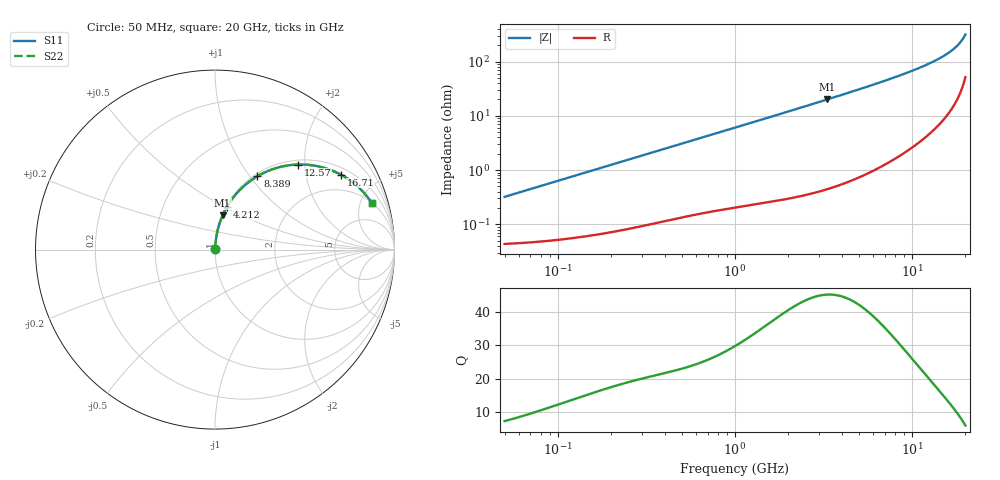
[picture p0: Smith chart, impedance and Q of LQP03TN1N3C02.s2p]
!Murata Part Number: LQP03TN1N3C02
!These Parameters are Measured in Series Mode Connection
!  o--[Z]--o
!Port1  Port2
!  o-------o
!Freq. Start=50[MHz] Stop=20[GHz], 401[Steps]
# Hz S RI R 50
!Freq.(Hz) S11(Real) S11(Imag) S21(Real) S21(Imag) S12(Real) S12(Imag) S22(Real) S22(Imag)
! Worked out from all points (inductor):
!   401 points, 50 MHz to 20 GHz, reference 50 ohm
!   read as one part in series: L = 1.01 nH near 51.52 MHz
!   highest Q = 45.1 at 3.314 GHz (marker M1), where L = 961 pH
!   S11 on the Smith chart (normalised r, x): 50 MHz: 1.00, +0.01; 4.212 GHz: 1.01, +0.51; 8.389 GHz: 1.04, +1.09; 12.57 GHz: 1.09, +1.85; 16.71 GHz: 1.27, +3.17; 20 GHz: 2.03, +6.23
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5e7  0.000445 0.00318  0.9996 -0.00318  0.9996 -0.00318  0.000445 0.00318
1.364002e8  0.00066 0.00858  0.9993 -0.00858  0.9993 -0.00858  0.00066 0.00858
3.721004e8  0.00161 0.0229  0.9984 -0.0229  0.9984 -0.0229  0.00161 0.0229
6.380365e8  0.00307 0.0387  0.9969 -0.0387  0.9969 -0.0387  0.00307 0.0387
1e9  0.00564 0.0599  0.9944 -0.0599  0.9944 -0.0599  0.00564 0.0599
1.714689e9  0.0131 0.1014  0.9869 -0.1014  0.9869 -0.1014  0.0131 0.1014
2.728004e9  0.0297 0.1587  0.9703 -0.1587  0.9703 -0.1587  0.0297 0.1587
3.314454e9  0.0424 0.1908  0.9576 -0.1908  0.9576 -0.1908  0.0424 0.1908
4.212059e9  0.0663 0.2378  0.9337 -0.2378  0.9337 -0.2378  0.0663 0.2378
5.683258e9  0.116 0.308  0.884 -0.308  0.884 -0.308  0.116 0.308
7.442007e9  0.1903 0.378  0.8097 -0.378  0.8097 -0.378  0.1903 0.378
8.389408e9  0.2358 0.4085  0.7642 -0.4085  0.7642 -0.4085  0.2358 0.4085
1.034674e10  0.3387 0.4537  0.6613 -0.4537  0.6613 -0.4537  0.3387 0.4537
1.257102e10  0.4646 0.4741  0.5354 -0.4741  0.5354 -0.4741  0.4646 0.4741
1.460232e10  0.5819 0.4624  0.4181 -0.4624  0.4181 -0.4624  0.5819 0.4624
1.573793e10  0.6469 0.4427  0.3531 -0.4427  0.3531 -0.4427  0.6469 0.4427
1.670968e10  0.7014 0.4176  0.2986 -0.4176  0.2986 -0.4176  0.7014 0.4176
1.747767e10  0.7437 0.392  0.2563 -0.392  0.2563 -0.392  0.7437 0.392
1.828096e10  0.7868 0.3588  0.2132 -0.3588  0.2132 -0.3588  0.7868 0.3588
1.88369e10  0.8159 0.3315  0.1841 -0.3315  0.1841 -0.3315  0.8159 0.3315
1.940974e10  0.845 0.2988  0.155 -0.2988  0.155 -0.2988  0.845 0.2988
2e10  0.8737 0.2594  0.1263 -0.2594  0.1263 -0.2594  0.8737 0.2594
